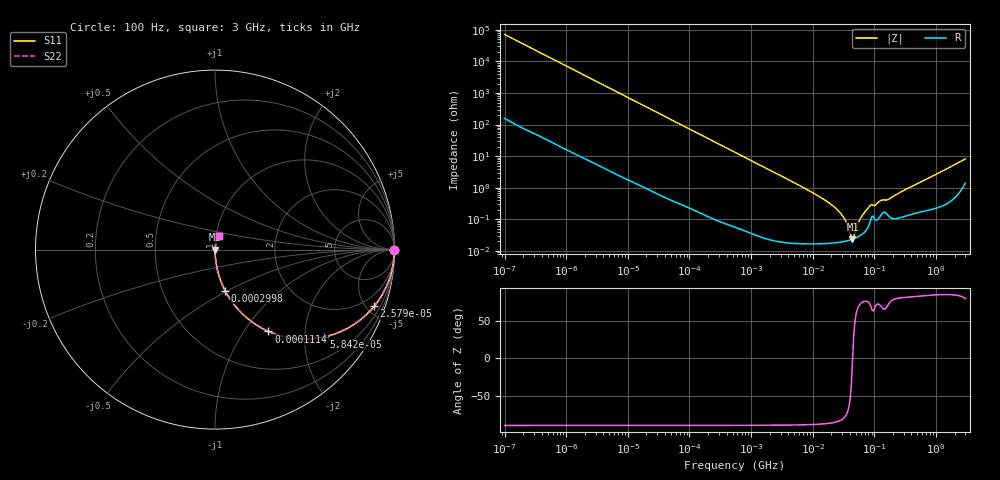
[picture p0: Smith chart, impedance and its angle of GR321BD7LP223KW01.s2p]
!Murata Part Number: GR321BD7LP223KW01
!These Parameters are Measured in Series Mode Connection
!Data Generated on Jan 08, 2026
!  o--ll--o
!Port1  Port2
!  o------o
!Operation Temp=25[degC], DC Bias Voltage=0[V]
!Freq. Start=100[Hz] Stop=3[GHz] 401[Steps]
# Hz S RI R 50
!Freq.(Hz) S11(Real) S11(Imag) S21(Real) S21(Imag) S12(Real) S12(Imag) S22(Real) S22(Imag)
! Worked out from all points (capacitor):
!   401 points, 100 Hz to 3 GHz, reference 50 ohm
!   read as one part in series: C = 22.2 nF near 109 Hz
!   lowest |Z| = 23.3 mohm at 44.18 MHz (marker M1)
!   series resonance near 44.37 MHz, so ESL is about 580 pH
!   S11 on the Smith chart (normalised r, x): 100 Hz: open; 25.79 kHz: 1.01, -5.61; 58.42 kHz: 1.01, -2.48; 111.4 kHz: 1.00, -1.30; 299.8 kHz: 1.00, -0.48; 3 GHz: 1.03, +0.16
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100  1 -0.00139  5e-06 0.00139  5e-06 0.00139  1 -0.00139
1788  0.9993 -0.0248  0.000673 0.0248  0.000673 0.0248  0.9993 -0.0248
8066  0.9874 -0.1103  0.0126 0.1103  0.0126 0.1103  0.9874 -0.1103
25785  0.8865 -0.3159  0.1135 0.3159  0.1135 0.3159  0.8865 -0.3159
31977  0.8359 -0.3691  0.1641 0.3691  0.1641 0.3691  0.8359 -0.3691
58416  0.6054 -0.4873  0.3946 0.4873  0.3946 0.4873  0.6054 -0.4873
111411  0.298 -0.4558  0.702 0.4558  0.702 0.4558  0.298 -0.4558
178874  0.1421 -0.3475  0.8579 0.3475  0.8579 0.3475  0.1421 -0.3475
299821  0.0561 -0.2284  0.9439 0.2284  0.9439 0.2284  0.0561 -0.2284
547723  0.0178 -0.1303  0.9822 0.1303  0.9822 0.1303  0.0178 -0.1303
9794414  0.000215 -0.00709  0.9998 0.00709  0.9998 0.00709  0.000215 -0.00709
1.789277e7  0.000183 -0.00342  0.9998 0.00342  0.9998 0.00342  0.000183 -0.00342
2.635803e7  0.000187 -0.0018  0.9998 0.0018  0.9998 0.0018  0.000187 -0.0018
3.268714e7  0.000199 -0.00103  0.9998 0.00103  0.9998 0.00103  0.000199 -0.00103
4.0536e7  0.00022 -0.000301  0.9998 0.000301  0.9998 0.000301  0.00022 -0.000301
4.418008e7  0.000232 -1.38e-05  0.9998 1.38e-05  0.9998 1.38e-05  0.000232 -1.38e-05
4.815176e7  0.000248 0.000275  0.9998 -0.000275  0.9998 -0.000275  0.000248 0.000275
5.9714e7  0.000309 0.00103  0.9997 -0.00103  0.9997 -0.00103  0.000309 0.00103
8.070971e7  0.000611 0.0023  0.9994 -0.0023  0.9994 -0.0023  0.000611 0.0023
1.295826e8  0.00141 0.00373  0.9986 -0.00373  0.9986 -0.00373  0.00141 0.00373
1.751444e8  0.00121 0.00424  0.9988 -0.00424  0.9988 -0.00424  0.00121 0.00424
3e9  0.02 0.0782  0.98 -0.0782  0.98 -0.0782  0.02 0.0782
